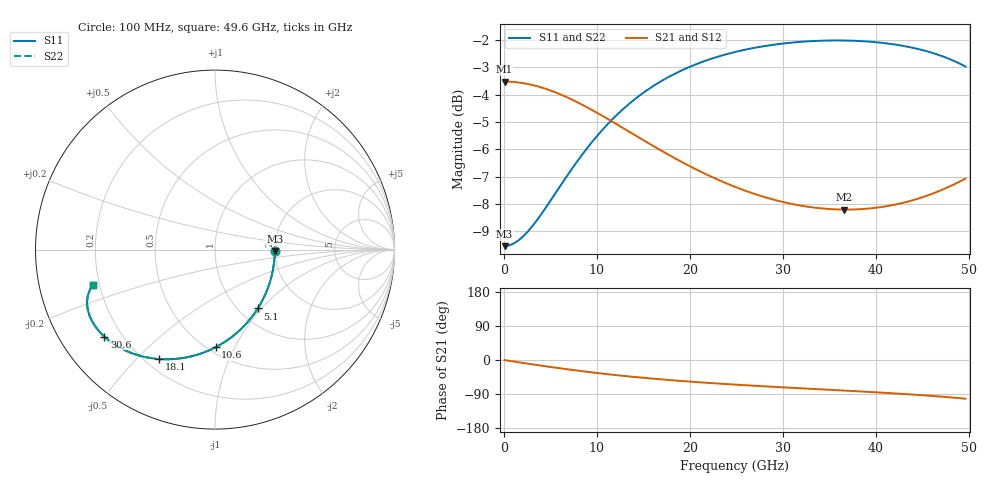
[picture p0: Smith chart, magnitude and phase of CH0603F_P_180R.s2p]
# GHz S RI R 180
! S-Parameters data
! Freq  reS11  imS11  reS21  imS21  reS12  imS12  reS22  imS22
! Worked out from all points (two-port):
!   100 points, 100 MHz to 49.6 GHz, reference 180 ohm
!   highest |S21| = -3.52 dB at 100 MHz (marker M1); lowest = -8.2 dB at 36.6 GHz (marker M2)
!   |S21| within 3 dB of the highest: start of sweep to 19.46 GHz
!   lowest |S11| = -9.5 dB at 100 MHz (marker M3), VSWR 2.00, Z = 360 - j5.63 ohm
!   |S11| at or under -10 dB: nowhere
!   |S22| runs from -9.5 to -2.0 dB; largest |S21 - S12| = 0
!   S11 on the Smith chart (normalised r, x): 100 MHz: 2.00, -0.03; 5.1 GHz: 1.22, -0.95; 10.6 GHz: 0.55, -0.84; 18.1 GHz: 0.25, -0.58; 30.6 GHz: 0.14, -0.34; 49.6 GHz: 0.17, -0.14
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0.1  0.3333 -0.00695  0.6666 -0.00435  0.6666 -0.00435  0.3333 -0.00695
1.1  0.3286 -0.0762  0.6637 -0.0477  0.6637 -0.0477  0.3286 -0.0762
2.6  0.3073 -0.1771  0.6504 -0.1108  0.6504 -0.1108  0.3073 -0.1771
3.6  0.2843 -0.2406  0.6361 -0.1503  0.6361 -0.1503  0.2843 -0.2406
5.1  0.2385 -0.3279  0.6079 -0.2046  0.6079 -0.2046  0.2385 -0.3279
7.1  0.1613 -0.4262  0.561 -0.2653  0.561 -0.2653  0.1613 -0.4262
8.6  0.0957 -0.4851  0.5218 -0.3015  0.5218 -0.3015  0.0957 -0.4851
10.6  0.00371 -0.5438  0.4676 -0.3381  0.4676 -0.3381  0.00371 -0.5438
12.1  -0.0654 -0.5744  0.4277 -0.3577  0.4277 -0.3577  -0.0654 -0.5744
13.6  -0.1327 -0.5948  0.3894 -0.3717  0.3894 -0.3717  -0.1327 -0.5948
16.6  -0.2569 -0.611  0.3201 -0.387  0.3201 -0.387  -0.2569 -0.611
18.1  -0.3127 -0.6095  0.2894 -0.3902  0.2894 -0.3902  -0.3127 -0.6095
21.6  -0.4253 -0.5895  0.2279 -0.3909  0.2279 -0.3909  -0.4253 -0.5895
25.1  -0.515 -0.5544  0.1784 -0.3872  0.1784 -0.3872  -0.515 -0.5544
27.6  -0.5666 -0.5242  0.1487 -0.3843  0.1487 -0.3843  -0.5666 -0.5242
30.6  -0.6167 -0.4847  0.1174 -0.3818  0.1174 -0.3818  -0.6167 -0.4847
33.1  -0.6498 -0.45  0.0939 -0.3813  0.0939 -0.3813  -0.6498 -0.45
36.6  -0.6843 -0.3996  0.0628 -0.3838  0.0628 -0.3838  -0.6843 -0.3996
41.6  -0.7103 -0.3246  0.0164 -0.3954  0.0164 -0.3954  -0.7103 -0.3246
45.6  -0.7093 -0.2622  -0.0293 -0.4121  -0.0293 -0.4121  -0.7093 -0.2622
47.6  -0.6994 -0.2305  -0.058 -0.4224  -0.058 -0.4224  -0.6994 -0.2305
49.6  -0.6816 -0.1994  -0.0928 -0.4332  -0.0928 -0.4332  -0.6816 -0.1994
